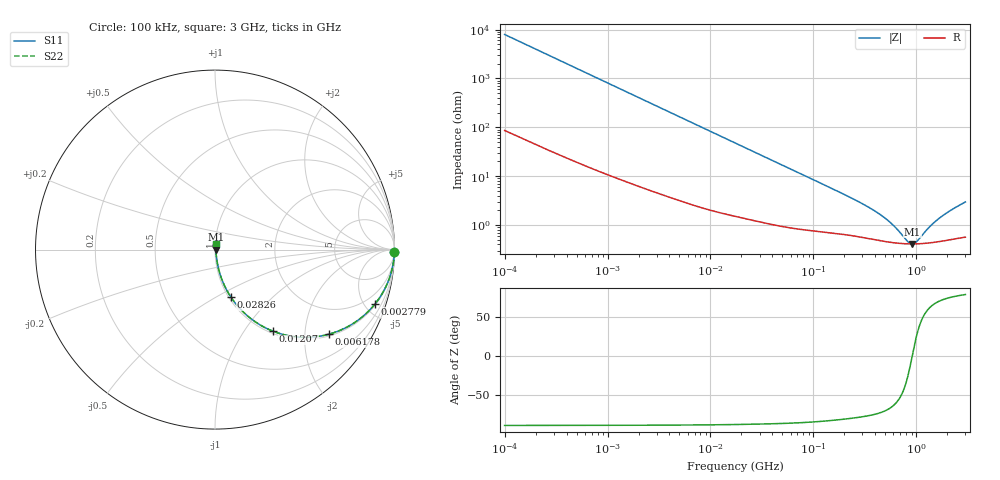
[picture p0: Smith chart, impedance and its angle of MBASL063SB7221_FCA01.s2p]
! MBASL063SB7221_FCA01  S-PARAMETER MODEL  ( Standard Model )
! Model Generated by TAIYO YUDEN Corporation (http://www.ty-top.com)
! Version 2.0
! TAIYO YUDEN Control No. 231201
! Copyright(c) 2020 TAIYO YUDEN CO.,LTD. All Rights Reserved.
! Product Description (link to TY-COMPAS)
! https://ds.yuden.co.jp/TYCOMPAS/or/detail?pn=MBASL063SB7221KFCA01&u=M
! Products Name : Multilayer Ceramic Capacitors
! Characteristics :
!  Capacitance : 220 [pF] , Rated Voltage : 10 [V] , TCC : X7R
!  Case Size : 0.6 x 0.3 / 0.024 x 0.012 [mm/inch] , Thickness : 0.3 / 0.012 [mm/inch]
!  (Conditions: Temperature = 25 [degC] , DC Bias Voltage = 0 [V])
! External Node Assignments :
!  1  o---| |---o  2
! GND o---------o GND
! Frequency Range : 100kHz  -  3GHz  [ 401 STEP ]
# MHZ S RI R 50
! Freq[MHz].  S11 Real  S11 Imag  S21 Real  S21 Imag  S12 Real  S12 Imag  S22 Real  S22 Imag
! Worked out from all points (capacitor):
!   401 points, 100 kHz to 3 GHz, reference 50 ohm
!   read as one part in series: C = 201 pF near 105.3 kHz
!   lowest |Z| = 411 mohm at 916.8 MHz (marker M1)
!   series resonance near 913.1 MHz, so ESL is about 150 pH
!   S11 on the Smith chart (normalised r, x): 100 kHz: open; 2.779 MHz: 1.10, -5.84; 6.178 MHz: 1.05, -2.65; 12.07 MHz: 1.04, -1.36; 28.26 MHz: 1.02, -0.59; 3 GHz: 1.01, +0.06
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0.1  0.9997 -0.0126  0.000297 0.0126  0.000297 0.0126  0.9997 -0.0126
0.562235  0.9943 -0.0697  0.00574 0.0697  0.00574 0.0697  0.9943 -0.0697
1.282589  0.9733 -0.1545  0.0267 0.1545  0.0267 0.1545  0.9733 -0.1545
2.778892  0.8911 -0.3034  0.1089 0.3034  0.1089 0.3034  0.8911 -0.3034
3.161081  0.8643 -0.334  0.1357 0.334  0.1357 0.334  0.8643 -0.334
6.178009  0.634 -0.4715  0.366 0.4715  0.366 0.4715  0.634 -0.4715
8.636841  0.4749 -0.488  0.5251 0.488  0.5251 0.488  0.4749 -0.488
12.07428  0.3218 -0.4541  0.6782 0.4541  0.6782 0.4541  0.3218 -0.4541
17.7727  0.1857 -0.3732  0.8143 0.3732  0.8143 0.3732  0.1857 -0.3732
28.26337  0.0889 -0.265  0.9111 0.265  0.9111 0.265  0.0889 -0.265
51.12795  0.0346 -0.1568  0.9654 0.1568  0.9654 0.1568  0.0346 -0.1568
97.38194  0.0148 -0.0844  0.9852 0.0844  0.9852 0.0844  0.0148 -0.0844
310.5665  0.00611 -0.0253  0.9939 0.0253  0.9939 0.0253  0.00611 -0.0253
423.1245  0.00514 -0.0168  0.9949 0.0168  0.9949 0.0168  0.00514 -0.0168
547.5153  0.00456 -0.0108  0.9954 0.0108  0.9954 0.0108  0.00456 -0.0108
826.9535  0.00411 -0.00202  0.9959 0.00202  0.9959 0.00202  0.00411 -0.00202
916.7529  0.00409 8.12e-05  0.9959 -8.12e-05  0.9959 -8.12e-05  0.00409 8.12e-05
1016.304  0.00411 0.00218  0.9959 -0.00218  0.9959 -0.00218  0.00411 0.00218
1349.411  0.00436 0.0081  0.9956 -0.0081  0.9956 -0.0081  0.00436 0.0081
1658.39  0.00471 0.0127  0.9953 -0.0127  0.9953 -0.0127  0.00471 0.0127
2201.951  0.00542 0.0197  0.9946 -0.0197  0.9946 -0.0197  0.00542 0.0197
3000  0.00644 0.0287  0.9936 -0.0287  0.9936 -0.0287  0.00644 0.0287
